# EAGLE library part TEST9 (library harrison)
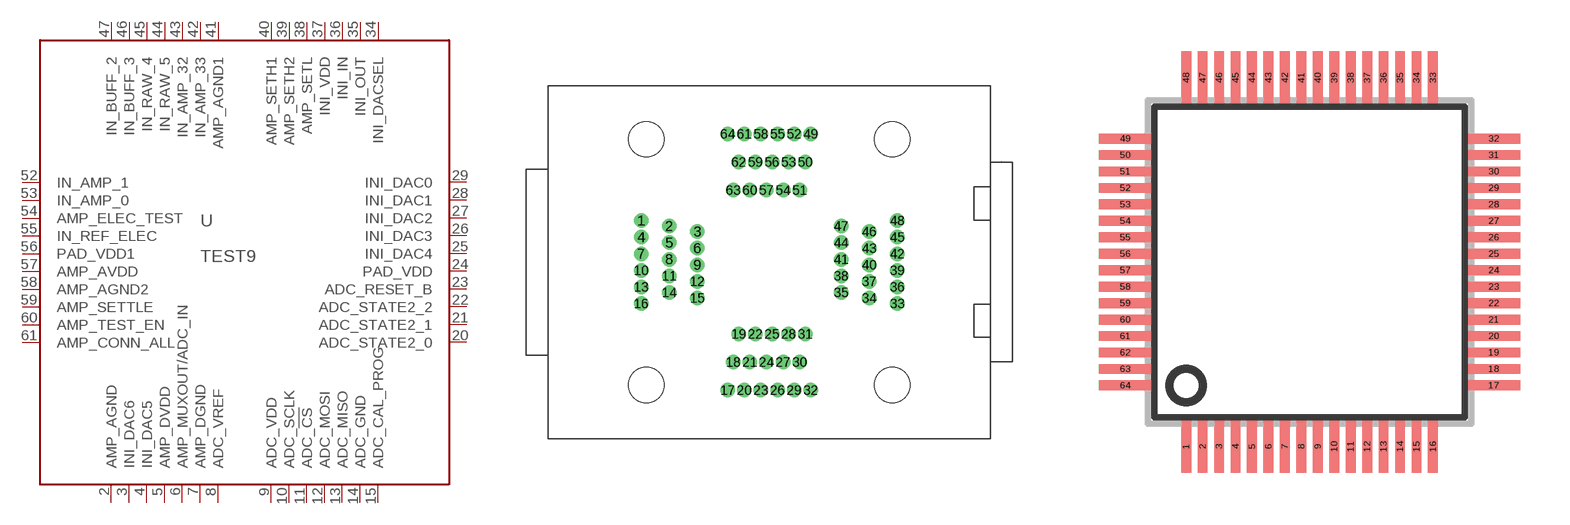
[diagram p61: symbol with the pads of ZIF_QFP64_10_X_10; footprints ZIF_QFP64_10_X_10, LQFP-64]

Designator prefix U

## TEST9  [ZIF_QFP64_10_X_10]
2  AMP_AGND  pwr
3  INI_DAC6  in
4  INI_DAC5  in
5  AMP_DVDD  pwr
6  AMP_MUXOUT/ADC_IN
7  AMP_DGND  pwr
8  ADC_VREF
9  ADC_VDD  pwr
10  ADC_SCLK  in
11  ADC_!CS!  in
12  ADC_MOSI  in
13  ADC_MISO  out
14  ADC_GND  pwr
15  ADC_CAL_PROG  out
20  ADC_STATE2_0  out
21  ADC_STATE2_1  out
22  ADC_STATE2_2  out
23  ADC_RESET_B  in
24  PAD_VDD  pwr
25  INI_DAC4  in
26  INI_DAC3  in
27  INI_DAC2  in
28  INI_DAC1  in
29  INI_DAC0  in
34  INI_DACSEL  in
35  INI_OUT  out
36  INI_IN  in
37  INI_VDD  pwr
38  AMP_SETL  pas
39  AMP_SETH2  pas
40  AMP_SETH1  pas
41  AMP_AGND1  pwr
42  IN_AMP_33  in
43  IN_AMP_32  in
44  IN_RAW_5  in
45  IN_RAW_4  in
46  IN_BUFF_3  in
47  IN_BUFF_2  in
52  IN_AMP_1  in
53  IN_AMP_0  in
54  AMP_ELEC_TEST  in
55  IN_REF_ELEC  in
56  PAD_VDD1  pwr
57  AMP_AVDD  pwr
58  AMP_AGND2  pwr
59  AMP_SETTLE  in
60  AMP_TEST_EN  in
61  AMP_CONN_ALL  in

## TEST9_QFP  [LQFP-64]
Pads as for ZIF_QFP64_10_X_10

## Footprint ZIF_QFP64_10_X_10 (pad centres in mm)
drill 0.8 pad 1.27: 1 -11.58,3.75; 2 -9.04,3.25; 3 -6.5,2.75; 4 -11.58,2.25; 5 -9.04,1.75; 6 -6.5,1.25; 7 -11.58,0.75; 8 -9.04,0.25; 9 -6.5,-0.25; 10 -11.58,-0.75; 11 -9.04,-1.25; 12 -6.5,-1.75; 13 -11.58,-2.25; 14 -9.04,-2.75; 15 -6.5,-3.25; 16 -11.58,-3.75; 17 -3.75,-11.58; 18 -3.25,-9.04; 19 -2.75,-6.5; 20 -2.25,-11.58; 21 -1.75,-9.04; 22 -1.25,-6.5; 23 -0.75,-11.58; 24 -0.25,-9.04; 25 0.25,-6.5; 26 0.75,-11.58; 27 1.25,-9.04; 28 1.75,-6.5; 29 2.25,-11.58; 30 2.75,-9.04; 31 3.25,-6.5; 32 3.75,-11.58; 33 11.58,-3.75; 34 9.04,-3.25; 35 6.5,-2.75; 36 11.58,-2.25; 37 9.04,-1.75; 38 6.5,-1.25; 39 11.58,-0.75; 40 9.04,-0.25; 41 6.5,0.25; 42 11.58,0.75; 43 9.04,1.25; 44 6.5,1.75; 45 11.58,2.25; 46 9.04,2.75; 47 6.5,3.25; 48 11.58,3.75; 49 3.75,11.58; 50 3.25,9.04; 51 2.75,6.5; 52 2.25,11.58; 53 1.75,9.04; 54 1.25,6.5; 55 0.75,11.58; 56 0.25,9.04; 57 -0.25,6.5; 58 -0.75,11.58; 59 -1.25,9.04; 60 -1.75,6.5; 61 -2.25,11.58; 62 -2.75,9.04; 63 -3.25,6.5; 64 -3.75,11.58
hole 3.2 at 11.1,11.1
hole 3.2 at -11.1,11.1
hole 3.2 at -11.1,-11.1
hole 3.2 at 11.1,-11.1

## Footprint LQFP-64 (pad centres in mm)
smd 0.3 x 1.6: 1 -3.75,-5.6; 2 -3.25,-5.6; 3 -2.75,-5.6; 4 -2.25,-5.6; 5 -1.75,-5.6; 6 -1.25,-5.6; 7 -0.75,-5.6; 8 -0.25,-5.6; 9 0.25,-5.6; 10 0.75,-5.6; 11 1.25,-5.6; 12 1.75,-5.6; 13 2.25,-5.6; 14 2.75,-5.6; 15 3.25,-5.6; 16 3.75,-5.6; 33 3.75,5.6; 34 3.25,5.6; 35 2.75,5.6; 36 2.25,5.6; 37 1.75,5.6; 38 1.25,5.6; 39 0.75,5.6; 40 0.25,5.6; 41 -0.25,5.6; 42 -0.75,5.6; 43 -1.25,5.6; 44 -1.75,5.6; 45 -2.25,5.6; 46 -2.75,5.6; 47 -3.25,5.6; 48 -3.75,5.6
smd 1.6 x 0.3: 17 5.6,-3.75; 18 5.6,-3.25; 19 5.6,-2.75; 20 5.6,-2.25; 21 5.6,-1.75; 22 5.6,-1.25; 23 5.6,-0.75; 24 5.6,-0.25; 25 5.6,0.25; 26 5.6,0.75; 27 5.6,1.25; 28 5.6,1.75; 29 5.6,2.25; 30 5.6,2.75; 31 5.6,3.25; 32 5.6,3.75; 49 -5.6,3.75; 50 -5.6,3.25; 51 -5.6,2.75; 52 -5.6,2.25; 53 -5.6,1.75; 54 -5.6,1.25; 55 -5.6,0.75; 56 -5.6,0.25; 57 -5.6,-0.25; 58 -5.6,-0.75; 59 -5.6,-1.25; 60 -5.6,-1.75; 61 -5.6,-2.25; 62 -5.6,-2.75; 63 -5.6,-3.25; 64 -5.6,-3.75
